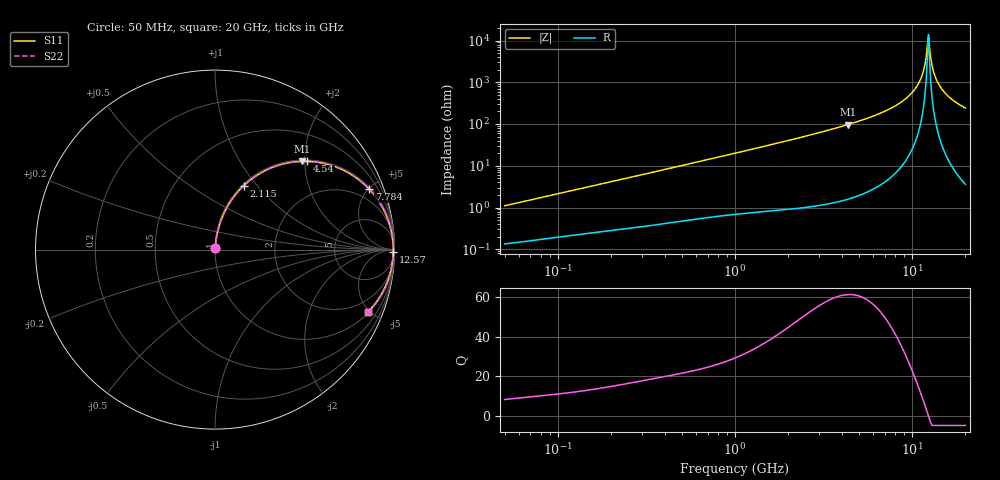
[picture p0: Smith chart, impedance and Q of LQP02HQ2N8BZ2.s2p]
!Murata Part Number: LQP02HQ2N8BZ2
!These Parameters are Measured in Series Mode Connection
!  o--[Z]--o
!Port1  Port2
!  o-------o
!Freq. Start=50[MHz] Stop=20[GHz], 401[Steps]
# Hz S RI R 50
!Freq.(Hz) S11(Real) S11(Imag) S21(Real) S21(Imag) S12(Real) S12(Imag) S22(Real) S22(Imag)
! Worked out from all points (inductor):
!   401 points, 50 MHz to 20 GHz, reference 50 ohm
!   read as one part in series: L = 3.45 nH near 51.52 MHz
!   highest Q = 61.2 at 4.34 GHz (marker M1), where L = 3.56 nH
!   self-resonance near 12.2 GHz
!   S11 on the Smith chart (normalised r, x): 50 MHz: 1.00, +0.02; 2.115 GHz: 1.02, +0.86; 4.54 GHz: 1.03, +2.06; 7.784 GHz: 1.12, +5.05; 12.57 GHz: open; 20 GHz: 1.07, -4.84
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5e7  0.00146 0.0109  0.9985 -0.0109  0.9985 -0.0109  0.00146 0.0109
1.364002e8  0.00312 0.0285  0.9969 -0.0285  0.9969 -0.0285  0.00312 0.0285
3.721004e8  0.00957 0.0747  0.9904 -0.0747  0.9904 -0.0747  0.00957 0.0747
1e9  0.0444 0.1896  0.9556 -0.1896  0.9556 -0.1896  0.0444 0.1896
2.114743e9  0.1603 0.3562  0.8397 -0.3562  0.8397 -0.3562  0.1603 0.3562
2.728004e9  0.2447 0.4206  0.7553 -0.4206  0.7553 -0.4206  0.2447 0.4206
4.34015e9  0.4851 0.4917  0.5149 -0.4917  0.5149 -0.4917  0.4851 0.4917
4.539627e9  0.5137 0.4917  0.4863 -0.4917  0.4863 -0.4917  0.5137 0.4917
7.442007e9  0.834 0.3614  0.166 -0.3614  0.166 -0.3614  0.834 0.3614
7.784049e9  0.8588 0.3369  0.1412 -0.3369  0.1412 -0.3369  0.8588 0.3369
9.316812e9  0.9402 0.2208  0.0598 -0.2208  0.0598 -0.2208  0.9402 0.2208
1.050288e10  0.975 0.1308  0.025 -0.1308  0.025 -0.1308  0.975 0.1308
1.098561e10  0.9834 0.0954  0.0166 -0.0954  0.0166 -0.0954  0.9834 0.0954
1.149051e10  0.9893 0.0593  0.0107 -0.0593  0.0107 -0.0593  0.9893 0.0593
1.166392e10  0.9906 0.0472  0.00937 -0.0472  0.00937 -0.0472  0.9906 0.0472
1.201863e10  0.9924 0.0229  0.00756 -0.0229  0.00756 -0.0229  0.9924 0.0229
1.220001e10  0.9929 0.0107  0.0071 -0.0107  0.0071 -0.0107  0.9929 0.0107
1.257102e10  0.9929 -0.0137  0.00709 0.0137  0.00709 0.0137  0.9929 -0.0137
1.334722e10  0.9893 -0.0624  0.0107 0.0624  0.0107 0.0624  0.9893 -0.0624
1.438523e10  0.9781 -0.1222  0.0219 0.1222  0.0219 0.1222  0.9781 -0.1222
1.646126e10  0.9402 -0.2242  0.0598 0.2242  0.0598 0.2242  0.9402 -0.2242
2e10  0.8505 -0.3492  0.1495 0.3492  0.1495 0.3492  0.8505 -0.3492
